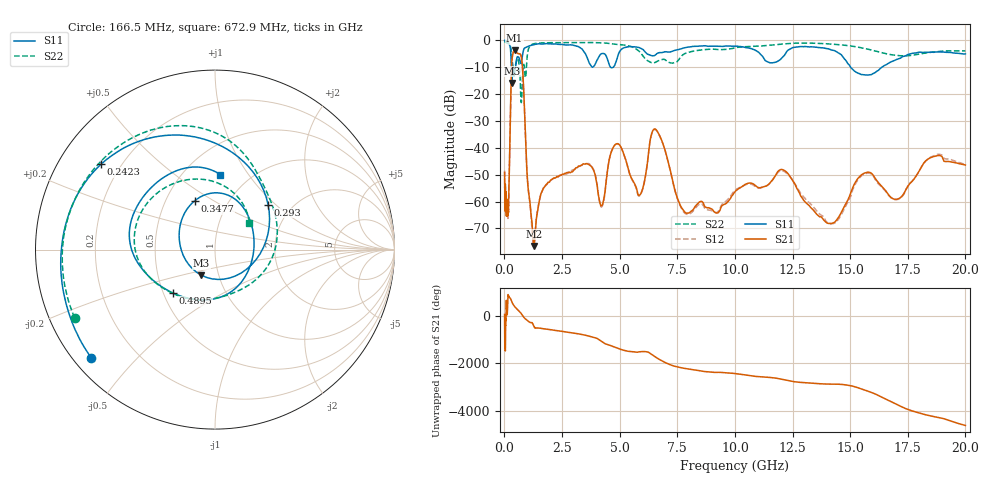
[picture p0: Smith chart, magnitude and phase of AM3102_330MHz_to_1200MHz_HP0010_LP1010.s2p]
! Date/Time: Tue, Sep 11, 2018 5:11 PM
! Network Analyzer: Agilent Technologies E8362B Rev: A.07.50.63
! Sweep from 0.010 to 20.000 GHz, 1601 Points, Sweep Type: LOG
! Power Supply: 4.949 V, 0.001 A
# Hz S DB R 50
!freq MagS11 AngS11 MagS21 AngS21 MagS12 AngS12 MagS22 AngS22
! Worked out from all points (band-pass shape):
!   1601 points, 10 MHz to 20 GHz, reference 50 ohm
!   highest |S21| = -3.69 dB at 445.1 MHz (marker M1); lowest = -76.6 dB at 1.29 GHz (marker M2)
!   |S21| within 3 dB of the highest: 334.8 MHz to 745.7 MHz (410.9 MHz wide, 76.1 % of centre)
!   lowest |S11| = -15.8 dB at 319.2 MHz (marker M3), VSWR 1.39, Z = 41.4 - j12.1 ohm
!   |S11| at or under -10 dB: 362.1 MHz to 481.6 MHz (119.5 MHz wide, 28.3 % of centre); 4.609 GHz to 4.72 GHz (110.8 MHz wide, 2.38 % of centre); 15.03 GHz to 16.38 GHz (1.353 GHz wide, 8.62 % of centre)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
!   |S22| runs from -23.2 to -0.3 dB; largest |S21 - S12| = 0.012
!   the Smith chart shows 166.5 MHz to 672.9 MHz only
!   S11 on the Smith chart (normalised r, x): 166.5 MHz: 0.05, -0.38; 242.3 MHz: 0.13, +0.33; 293 MHz: 1.52, +0.90; 347.7 MHz: 0.70, +0.41; 489.5 MHz: 0.56, -0.31; 672.9 MHz: 0.74, +0.75
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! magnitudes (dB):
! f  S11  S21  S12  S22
! 10 MHz  0.0  -49.2  -48.5  -0.3
! 35.55 MHz  0.0  -61.0  -60.6  -0.5
! 126.4 MHz  -0.4  -62.8  -62.4  -1.0
! 166.5 MHz  -0.8  -63.4  -65.2  -1.2
! 242.3 MHz  -2.0  -36.4  -36.5  -1.8
! 293 MHz  -8.2  -15.0  -15.1  -3.6
! 319.2 MHz  -15.8  -8.4  -8.4  -6.1
! 347.7 MHz  -10.6  -5.9  -6.0  -8.2
! 445.1 MHz  -12.0  -3.7  -3.7  -10.6
! 447.2 MHz  -11.9  -3.7  -3.7  -10.5
! 489.5 MHz  -9.5  -3.8  -3.9  -8.7
! 672.9 MHz  -7.6  -5.0  -5.0  -12.3
! 1.29 GHz  -1.6  -76.6  -75.8  -1.2
! 1.59 GHz  -1.3  -57.1  -57.0  -0.9
! 4.21 GHz  -5.0  -61.5  -62.0  -0.9
! 4.878 GHz  -7.1  -38.5  -38.5  -1.5
! 5.652 GHz  -2.4  -53.4  -53.7  -2.9
! 6.58 GHz  -5.2  -33.3  -33.4  -8.0
! 7.882 GHz  -2.6  -64.3  -64.6  -4.7
! 12.03 GHz  -6.6  -48.0  -48.5  -1.4
! 14.14 GHz  -3.4  -68.1  -68.5  -1.3
! 20 GHz  -5.0  -46.4  -46.3  -3.9
